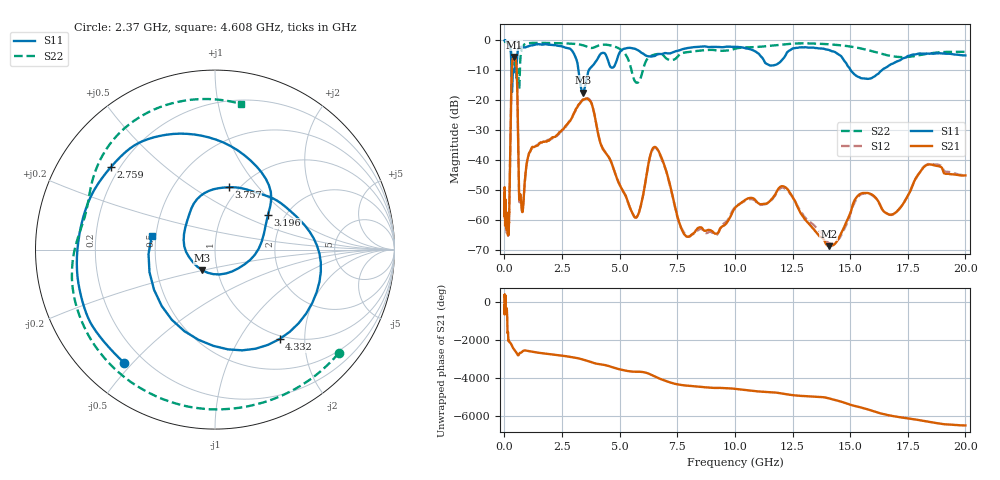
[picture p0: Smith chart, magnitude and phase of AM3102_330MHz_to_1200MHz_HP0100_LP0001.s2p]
! Date/Time: Tue, Sep 11, 2018 5:12 PM
! Network Analyzer: Agilent Technologies E8362B Rev: A.07.50.63
! Sweep from 0.010 to 20.000 GHz, 1601 Points, Sweep Type: LOG
! Power Supply: 4.949 V, 0.001 A
# Hz S DB R 50
!freq MagS11 AngS11 MagS21 AngS21 MagS12 AngS12 MagS22 AngS22
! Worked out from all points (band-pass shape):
!   1601 points, 10 MHz to 20 GHz, reference 50 ohm
!   highest |S21| = -5.54 dB at 414.5 MHz (marker M1); lowest = -68.7 dB at 14.07 GHz (marker M2)
!   |S21| within 3 dB of the highest: 330.4 MHz to 524.6 MHz (194.2 MHz wide, 45.4 % of centre)
!   lowest |S11| = -17.4 dB at 3.416 GHz (marker M3), VSWR 1.31, Z = 42.3 - j9.87 ohm
!   |S11| at or under -10 dB: 308 MHz to 366.9 MHz (58.91 MHz wide, 17.5 % of centre); 3.212 GHz to 3.661 GHz (449.1 MHz wide, 13.1 % of centre); 15.03 GHz to 16.37 GHz (1.342 GHz wide, 8.55 % of centre)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
!   |S22| runs from -16.2 to -0.2 dB; largest |S21 - S12| = 0.0069
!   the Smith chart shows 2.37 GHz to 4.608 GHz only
!   S11 on the Smith chart (normalised r, x): 2.37 GHz: 0.13, -0.47; 2.759 GHz: 0.17, +0.34; 3.196 GHz: 1.64, +0.73; 3.757 GHz: 0.90, +0.71; 4.332 GHz: 0.94, -1.51; 4.608 GHz: 0.47, +0.08
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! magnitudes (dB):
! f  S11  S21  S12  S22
! 10 MHz  0.0  -49.4  -49.0  -0.2
! 35.55 MHz  0.0  -58.5  -59.3  -0.4
! 126.4 MHz  -0.4  -62.8  -62.1  -0.8
! 200.4 MHz  -1.2  -60.6  -60.9  -1.3
! 319.2 MHz  -15.1  -10.7  -10.7  -7.3
! 414.5 MHz  -10.7  -5.5  -5.6  -7.6
! 447.2 MHz  -9.6  -5.8  -5.8  -7.2
! 765 MHz  -2.3  -56.9  -57.1  -2.4
! 1.59 GHz  -1.4  -34.0  -34.1  -0.8
! 2.37 GHz  -1.8  -30.8  -31.2  -0.9
! 2.759 GHz  -2.6  -27.7  -27.8  -1.0
! 3.196 GHz  -9.0  -21.6  -21.9  -1.3
! 3.416 GHz  -17.4  -19.7  -19.9  -1.6
! 3.757 GHz  -9.0  -20.6  -20.6  -2.5
! 4.332 GHz  -4.2  -36.9  -36.8  -1.4
! 4.608 GHz  -8.9  -40.1  -40.1  -1.7
! 5.652 GHz  -2.8  -59.0  -58.9  -13.5
! 6.58 GHz  -4.9  -35.8  -36.0  -4.6
! 7.92 GHz  -2.6  -65.5  -65.4  -3.9
! 12.09 GHz  -6.1  -48.7  -49.2  -1.3
! 14.07 GHz  -3.2  -68.7  -67.6  -1.3
! 20 GHz  -5.0  -45.1  -45.2  -3.8
